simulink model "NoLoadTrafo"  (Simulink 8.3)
settings: Solver=ode23s  StartTime=0.0  StopTime=30  MaxStep=0.5e-3  RelTol=1e-6
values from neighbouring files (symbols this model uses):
  I0 = interp1(s,abs(I1),0)    [Ex7i_IM.m]    (also in Psi2I0.m = pi*poles*Ftot/(2*nphase*N1*fw))
  kl = 0:0.01:klmax; kl(1)=1e-4    [Ex2_trFunc.m]
  L1sig = din(6)    [Ex7i_IM.m]
  R1 = Rsc*R1perR2/(1+R1perR2)    [Ex2_trFunc.m]    (also in Ex7i_IM.m = din(4); Ex8i_SM.m = r_1*Xb; im1_ohg.m = 76.640326; im1_oga.m = 80.165355)
undefined symbols (not defined in the file or in its folder): Imref, Lmtrref

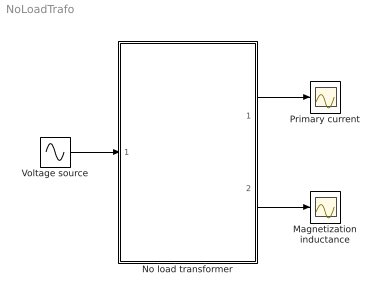
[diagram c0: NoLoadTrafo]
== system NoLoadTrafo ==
  Magnetization inductance : Scope
  No load transformer : Subsystem
  Primary current : Scope
  Voltage source : Sin  Amplitude=400*sqrt(2)  Frequency=100*pi  SampleTime=0
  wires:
  Voltage source/1 -> No load transformer/1("V1 ")
  No load transformer/1(i1) -> Primary current/1
  No load transformer/2(Lm) -> Magnetization inductance/1

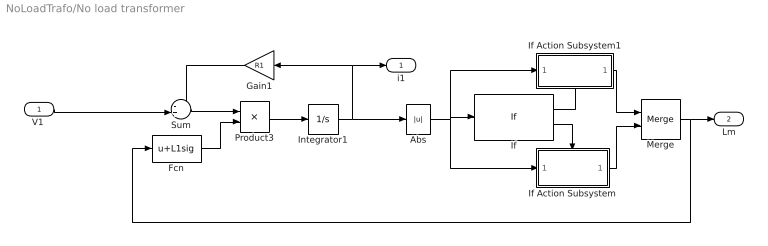
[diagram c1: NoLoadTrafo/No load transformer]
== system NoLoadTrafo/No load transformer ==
  "V1 " : Inport
  Abs : Abs
  Fcn : Fcn  Expr=u+L1sig
  Gain1 : Gain  Gain=R1
  If : If  IfExpression=u1 < I0max
  If Action Subsystem : Subsystem  TreatAsAtomicUnit=on
  If Action Subsystem1 : Subsystem  TreatAsAtomicUnit=on
  Integrator1 : Integrator
  Merge : Merge
  Product3 : Product  Inputs=*/
  Sum : Sum  Inputs=-+|
  i1 : Outport
  Lm : Outport  Port=2
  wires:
  "V1 "/1 -> Sum/2
  Gain1/1 -> Sum/1
  Sum/1 -> Product3/1
  Fcn/1 -> Product3/2
  Abs/1 -> If/1, If Action Subsystem/1(In1), If Action Subsystem1/1(In1)
  If/2 -> If Action Subsystem/Action
  If/1 -> If Action Subsystem1/Action
  If Action Subsystem1/1(Out1) -> Merge/1
  If Action Subsystem/1(Out1) -> Merge/2
  Merge/1 -> Lm/1, Fcn/1
  Integrator1/1 -> Gain1/1, i1/1, Abs/1
  Product3/1 -> Integrator1/1

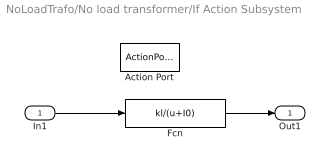
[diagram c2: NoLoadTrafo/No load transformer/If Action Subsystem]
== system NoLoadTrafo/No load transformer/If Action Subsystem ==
  In1 : Inport
  Action Port : ActionPort  ActionType=else
  Fcn : Fcn  Expr=kl/(u+I0)
  Out1 : Outport
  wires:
  In1/1 -> Fcn/1
  Fcn/1 -> Out1/1

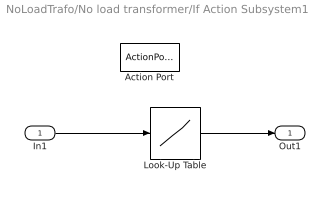
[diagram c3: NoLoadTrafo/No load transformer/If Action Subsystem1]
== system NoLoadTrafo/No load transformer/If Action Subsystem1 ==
  In1 : Inport
  Action Port : ActionPort  ActionType=then
  Look-Up Table : Lookup  InputValues=Imref  Table=Lmtrref
  Out1 : Outport
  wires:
  In1/1 -> Look-Up Table/1
  Look-Up Table/1 -> Out1/1
